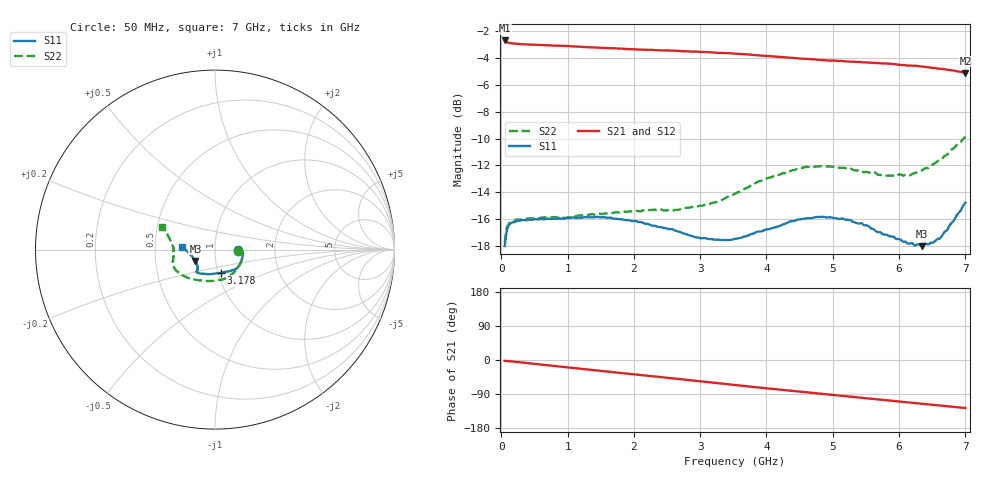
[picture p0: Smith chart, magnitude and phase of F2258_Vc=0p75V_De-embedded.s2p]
! Integrated Device Technology
! Corporate Headquarters
! 6024 Silver Creek Valley Road
! San Jose, CA 95138  USA
! Phone:  1-408-284-8200
! Toll Free:  1-800-223-1366
! Webpage:  http://www.idt.com/
! Timing and RF Division
! 515 Groton Road, Suite 102
! Westford, MA 01886-6024
! Device:  F2258
! Description: Voltage Variable RF Attenuator
! Frequency:  50.0 -  6000.00 MHz
! Package:  3x3 mm Thin QFN Plastic Package: 16 pin
! Ports:  2 RF, 2 DC
!  Pin  1  = NC
!  Pin  2  = NC
!  Pin  3  = RF2  = Port 2
!  Pin  4  = GND
!  Pin  5  = Vdd
!  Pin  6  = NC
!  Pin  7  = VCTRL
!  Pin  8  = NC
!  Pin  9  = GND
!  Pin 10  = RF1  = Port 1
!  Pin 11  = NC
!  Pin 12  = NC
!  Pin 13  = NC
!  Pin 14  = NC
!  Pin 15  = NC
!  Pin 16  = NC
! Vcntrl:  0.750 Volts
! Vdd:  +3.300 Volts
! Current:  1.127 mA
! Data:  The device was measured on a the F2258 evaluation board which has
!  individual transmission lines to the RF pins.  Data was collected
!  using a calibrated network analyzer.  The evaluation board was
!  de-embedded using a TRL calibration technique.
!  The reference plane is the edge of the package pin.
! Misc:  SN 10
!  Action Tracker AT0285
! Date Measured:  2014-12-10
! Date:  2016-01-13  MJV
! Note:
!  Integrated Device Technology supplies this data as a sample of measured
!  data at the package pin for this product.  Your particular data for this
!  product may vary.
!  Data was taken at 25 degrees C.
!  Integrated Device Technology reserves the right to change this data at anytime.
!Freq_(GHz)  S11M_(dB)  S11P_(deg)  S21M_(dB)  S21P_(deg)  S12M_(dB)  S12P_(deg)  S22M_(dB)  S22P_(deg)
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# GHz S dB R 50
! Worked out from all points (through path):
!   201 points, 50 MHz to 7 GHz, reference 50 ohm
!   highest |S21| = -2.71 dB at 50 MHz (marker M1); lowest = -5.1 dB at 7 GHz (marker M2)
!   group delay of S21, straight-line fit = 50.1 ps
!   lowest |S11| = -18.0 dB at 6.34 GHz (marker M3), VSWR 1.29, Z = 39.9 - j5.13 ohm
!   |S11| at or under -10 dB: start of sweep to end of sweep
!   |S22| runs from -17.7 to -9.9 dB; largest |S21 - S12| = 0.0024
!   S11 on the Smith chart (normalised r, x): 50 MHz: 1.29, -0.01; 3.178 GHz: 1.03, -0.27; 7 GHz: 0.69, +0.02
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0.05  -17.99 -2.1  -2.71 -2.1  -2.72 -2.2  -17.71 -2.8
0.08475  -16.76 -2.9  -2.84 -2.6  -2.86 -2.6  -16.57 -3.6
0.15425  -16.25 -4.3  -2.92 -3.7  -2.94 -3.7  -16.16 -6.4
0.606  -15.97 -16.4  -3.04 -12.2  -3.07 -12.2  -15.87 -23.2
0.9535  -15.92 -26.4  -3.12 -18.7  -3.13 -18.7  -15.93 -36.9
1.2315  -15.87 -32.2  -3.19 -23.9  -3.21 -23.9  -15.70 -46.3
1.6485  -15.87 -39.7  -3.29 -31.4  -3.29 -31.4  -15.54 -58.9
2.37825  -16.57 -51.5  -3.43 -44.6  -3.44 -44.6  -15.31 -78.9
2.58675  -16.75 -56.2  -3.47 -48.4  -3.48 -48.4  -15.36 -85.3
2.93425  -17.35 -66.2  -3.53 -54.8  -3.55 -54.8  -15.11 -97.6
3.1775  -17.48 -75.1  -3.60 -59.4  -3.61 -59.4  -14.80 -107.0
3.525  -17.46 -90.5  -3.69 -65.9  -3.70 -65.9  -14.10 -121.1
4.0115  -16.74 -110.9  -3.86 -75.0  -3.87 -75.0  -12.94 -138.3
4.498  -16.01 -123.6  -4.06 -83.7  -4.06 -83.7  -12.19 -151.2
4.7065  -15.89 -126.2  -4.11 -87.3  -4.11 -87.3  -12.13 -155.3
4.8455  -15.81 -127.6  -4.17 -89.8  -4.16 -89.8  -12.03 -157.7
5.2625  -16.05 -130.5  -4.29 -96.8  -4.30 -96.8  -12.19 -164.5
5.85325  -17.27 -135.1  -4.44 -106.9  -4.45 -107.0  -12.75 -175.8
6.166  -17.80 -141.9  -4.57 -112.4  -4.56 -112.4  -12.73 177.3
6.33975  -18.00 -149.8  -4.64 -115.5  -4.64 -115.5  -12.39 172.5
6.61775  -17.44 -166.1  -4.82 -120.3  -4.79 -120.3  -11.60 165.4
7  -14.78 175.0  -5.12 -126.6  -5.09 -126.6  -9.86 157.1
